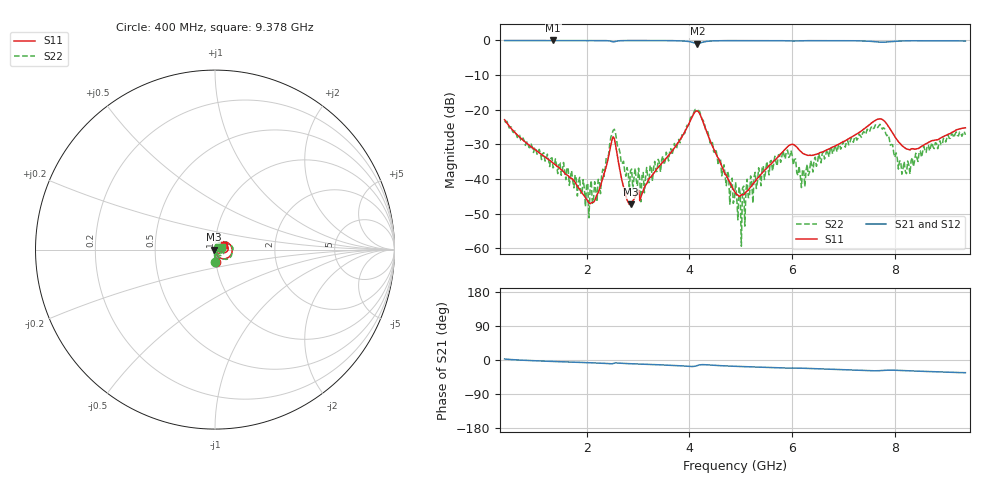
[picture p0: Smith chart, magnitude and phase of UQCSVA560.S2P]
!  Part Number  UQCSVA560  Mounting Orientation: Horizontal
!  Description: Ultra Low ESR Microwave capacitors
!  Application: Coupling, Bypass, Tuning, DC Block
!  Filters, Matching
# GHZ S DB R 50
! Freq  |S11|  S11 Ph  |S21|  S21 Ph  |S12|  S12 Ph  |S22|  S22 Ph
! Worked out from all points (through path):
!   400 points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, 400 MHz to 9.378 GHz, reference 50 ohm
!   highest |S21| = -0.01 dB at 1.345 GHz (marker M1); lowest = -0.9 dB at 4.158 GHz (marker M2)
!   group delay of S21, straight-line fit = 10.2 ps
!   lowest |S11| = -47.3 dB at 2.853 GHz (marker M3), VSWR 1.01, Z = 49.6 - j0.0732 ohm
!   |S11| at or under -10 dB: start of sweep to end of sweep
!   |S22| runs from -59.4 to -19.9 dB; largest |S21 - S12| = 0.0043
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0.4  -22.89 -86.3  -0.03 2.7  -0.02 2.7  -23.27 -89.1
1.345  -35.40 -98.9  -0.01 -3.9  -0.01 -3.9  -36.77 -97.7
1.908  -44.02 -135.6  -0.01 -6.5  0.00 -6.5  -44.19 -41.5
2.2  -44.49 134.7  -0.02 -8.0  -0.01 -8.0  -46.54 19.7
2.515  -27.80 8.4  -0.42 -9.2  -0.41 -9.3  -25.96 -8.0
2.853  -47.31 -170.1  -0.03 -9.8  -0.02 -9.9  -37.63 -17.7
3.01  -43.23 143.4  -0.02 -10.6  -0.01 -10.7  -36.84 0.2
3.055  -45.14 105.8  -0.02 -10.9  -0.01 -10.9  -46.54 19.9
3.393  -36.62 82.1  -0.04 -12.6  -0.03 -12.7  -34.31 43.4
4.158  -20.37 -10.9  -0.90 -14.5  -0.90 -14.6  -20.29 -13.3
4.788  -40.95 -61.7  -0.06 -16.1  -0.05 -16.2  -47.24 -65.7
4.9  -44.05 -40.7  -0.04 -16.7  -0.04 -16.8  -40.90 -28.8
4.945  -44.60 -29.7  -0.05 -16.9  -0.04 -17.0  -51.77 43.2
4.99  -44.93 -16.8  -0.05 -17.1  -0.04 -17.2  -44.26 -34.8
5.013  -44.51 -11.4  -0.04 -17.2  -0.04 -17.4  -59.35 58.7
5.035  -44.51 -7.6  -0.04 -17.3  -0.04 -17.5  -42.65 43.3
5.08  -44.14 4.3  -0.04 -17.6  -0.04 -17.7  -53.56 -8.1
5.125  -43.42 11.1  -0.04 -17.8  -0.04 -17.9  -40.05 31.7
6.408  -33.10 20.8  -0.06 -22.7  -0.06 -22.8  -37.97 79.2
7.893  -25.11 -17.9  -0.40 -26.8  -0.40 -26.9  -28.24 -30.7
8.298  -31.59 6.6  -0.10 -28.7  -0.12 -28.8  -38.56 26.5
9.378  -25.21 25.6  -0.18 -33.5  -0.20 -33.6  -27.24 21.9
